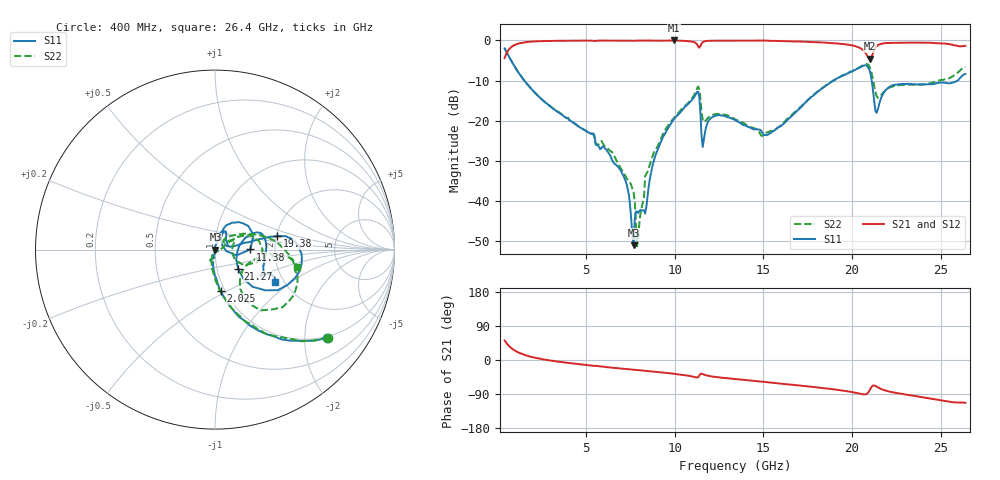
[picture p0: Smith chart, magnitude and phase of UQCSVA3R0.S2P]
!  Part Number  UQCSVA3R0  Mounting Orientation: Horizontal
!  Description: Ultra Low ESR Microwave capacitors
!  Application: Coupling, Bypass, Tuning, DC Block
!  Filters, Matching
# GHZ S DB R 50
! Freq  |S11|  S11 Ph  |S21|  S21 Ph  |S12|  S12 Ph  |S22|  S22 Ph
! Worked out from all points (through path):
!   401 points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, 400 MHz to 26.4 GHz, reference 50 ohm
!   highest |S21| = 0.00 dB at 9.955 GHz (marker M1); lowest = -4.6 dB at 21 GHz (marker M2)
!   group delay of S21, straight-line fit = 13.3 ps
!   lowest |S11| = -51.2 dB at 7.68 GHz (marker M3), VSWR 1.01, Z = 50.3 - j0.109 ohm
!   |S11| at or under -10 dB: 1.505 GHz to 18.96 GHz (17.46 GHz wide, 171 % of centre); 21.11 GHz to 25.95 GHz (4.841 GHz wide, 20.6 % of centre)
!   |S22| runs from -51.4 to -2.0 dB; largest |S21 - S12| = 0.011
!   S11 on the Smith chart (normalised r, x): 400 MHz: 0.96, -2.57; 2.025 GHz: 0.96, -0.47; 11.38 GHz: 1.49, +0.00; 19.38 GHz: 2.03, +0.35; 21.27 GHz: 1.26, -0.28; 26.4 GHz: 1.81, -0.76
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0.4  -1.99 -38.3  -4.41 51.5  -4.41 51.5  -1.97 -38.0
1.05  -7.09 -66.6  -0.96 22.9  -0.98 22.9  -7.13 -66.6
2.025  -12.65 -82.0  -0.26 6.9  -0.27 6.8  -12.66 -83.0
4.755  -21.94 -97.1  -0.05 -11.9  -0.06 -12.0  -21.97 -103.6
7.03  -33.15 -98.4  -0.04 -22.8  -0.04 -22.8  -32.44 -111.8
7.68  -51.16 -23.1  -0.08 -25.7  -0.09 -25.7  -37.96 -111.3
7.94  -43.07 -6.2  -0.03 -26.7  -0.04 -26.8  -49.31 -27.8
8.46  -39.12 110.5  -0.03 -29.3  -0.03 -29.3  -32.80 -15.9
9.11  -26.45 73.7  -0.07 -32.2  -0.06 -32.2  -25.73 21.2
9.955  -19.57 69.8  0.00 -36.4  -0.02 -36.4  -19.41 29.2
11.19  -13.43 43.7  -0.65 -45.9  -0.66 -45.9  -12.67 17.0
11.385  -14.11 0.2  -1.82 -40.9  -1.79 -40.8  -12.18 -16.2
11.645  -24.63 54.3  -0.28 -38.5  -0.28 -38.5  -20.41 -3.1
12.165  -18.98 62.9  -0.06 -43.9  -0.07 -44.0  -18.55 22.5
13.4  -19.86 51.6  -0.06 -50.3  -0.08 -50.3  -19.68 29.0
15.22  -23.58 18.4  -0.07 -58.9  -0.07 -59.0  -22.96 47.4
17.755  -13.96 12.6  -0.40 -70.7  -0.40 -70.7  -13.83 25.9
19.38  -8.98 12.1  -0.86 -80.1  -0.86 -80.1  -8.98 5.1
21.005  -7.59 -32.8  -4.58 -79.5  -4.55 -78.9  -6.70 -46.1
21.265  -15.56 -39.5  -2.32 -67.3  -2.34 -67.4  -11.71 -57.2
22.11  -11.60 21.0  -0.63 -83.3  -0.64 -83.3  -11.81 -9.8
26.4  -8.37 -28.1  -1.34 -113.2  -1.34 -113.2  -6.58 -12.2
